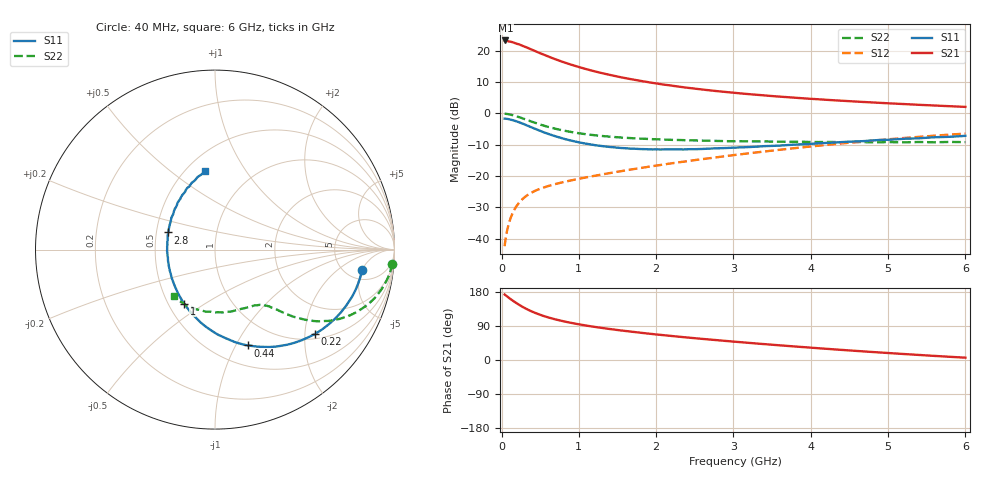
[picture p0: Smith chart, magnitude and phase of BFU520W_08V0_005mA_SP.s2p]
! Filename:  P:\Prog\Test\Noise\ATS_data\Testdata_Net\Run2\BFU520W_APM2013_06_A05_08p0V_005mA_SP_CM01_D.s2p
! Date/Time: Tue 26/Mar/2013 18:01:42
! BFU520W_APM2013_06_A05_08p0V_1to20mA_SP_CM01_Bias4_R.s2p
! MDIF S-parameter v. bias file
! BFU520W_APM2013_06_A05_08p0V_1to20mA_SP_CM01
! Date/time Thu Mar 21 15:28:29 2013
! VAR V_out= 8.0000
! VAR I_out= 4.9950
! VAR V_in= 0.8219
! VAR I_in= 0.0543
! Device data file deembeded for feedlines and parallel
! Original file: \Run2\BFU520W_APM2013_06_A05_08p0V_005mA_SP_CM01_R.s2p
! Feed-files: PR019V01_070313_Feed1.s2p, PR019V01_070313_Feed2.s2p
! Parallel-file: PR019V01_070313_Par.s2p
# MHz S MA R 50
!  Freq-MHz  S11-mag  S11-arg  S21-mag  S21-arg  S12-mag  S12-arg  S22-mag  S22-arg
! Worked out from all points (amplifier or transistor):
!   98 points, 40 MHz to 6 GHz, reference 50 ohm
!   highest |S21| = 23.3 dB at 50 MHz (marker M1)
!   |S21| within 3 dB of that: start of sweep to 398.1 MHz
!   unconditionally stable (mu >= 1): 1.86 GHz to 3.015 GHz
!   at 300 MHz: K = 0.33, MSG = 24.0 dB, |S12| = -26.7 dB
!   at 1.6 GHz: K = 0.97, MSG = 14.7 dB, |S12| = -18.2 dB
!   at 6 GHz: K = 0.86, MSG = 4.3 dB, |S12| = -6.4 dB
!   S11 on the Smith chart (normalised r, x): 40 MHz: 7.00, -5.01; 220 MHz: 1.12, -2.24; 440 MHz: 0.72, -1.12; 1 GHz: 0.60, -0.41; 2.8 GHz: 0.58, +0.12; 6 GHz: 0.62, +0.67
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40  0.8281 -7.8  14.61 173.0  0.007608 85.1  0.9909 -4.5
50  0.8258 -9.7  14.62 171.3  0.009427 84.6  0.9883 -5.6
60  0.8224 -11.6  14.4 169.6  0.01126 83.6  0.9852 -6.8
120  0.7952 -23.0  13.98 160.3  0.02175 77.8  0.955 -13.2
140  0.7837 -26.6  13.73 157.4  0.02499 76.0  0.9413 -15.2
220  0.7281 -40.3  12.75 146.6  0.03664 69.8  0.8784 -22.2
260  0.6976 -46.5  12.19 141.7  0.04163 67.2  0.8454 -25.2
320  0.6501 -55.5  11.4 135.0  0.04812 64.1  0.7948 -29.0
380  0.6058 -63.5  10.57 129.2  0.05366 61.6  0.7472 -32.1
440  0.5648 -71.0  9.843 124.0  0.0586 59.8  0.7052 -34.5
550  0.4976 -83.0  8.644 115.8  0.06596 57.6  0.6368 -37.9
700  0.4311 -97.1  7.311 107.0  0.07479 56.4  0.5688 -40.8
850  0.3816 -109.2  6.293 100.0  0.08277 56.2  0.5194 -42.6
1000  0.3463 -119.9  5.513 94.2  0.09048 56.7  0.4832 -44.0
1050  0.3369 -123.1  5.288 92.4  0.09299 56.9  0.4736 -44.5
1450  0.2886 -146.6  4.002 80.5  0.1144 58.7  0.421 -47.7
2050  0.266 -174.1  2.949 66.5  0.15 60.4  0.3849 -53.8
2800  0.2781 159.8  2.263 52.1  0.2008 60.3  0.3639 -64.3
3100  0.2876 151.3  2.084 46.9  0.2234 59.5  0.36 -68.9
4100  0.3334 128.8  1.683 31.0  0.3057 54.9  0.3491 -87.6
5200  0.3934 109.3  1.413 15.8  0.4048 46.6  0.3458 -111.6
6000  0.4388 97.3  1.272 6.1  0.4768 39.2  0.3481 -131.4
